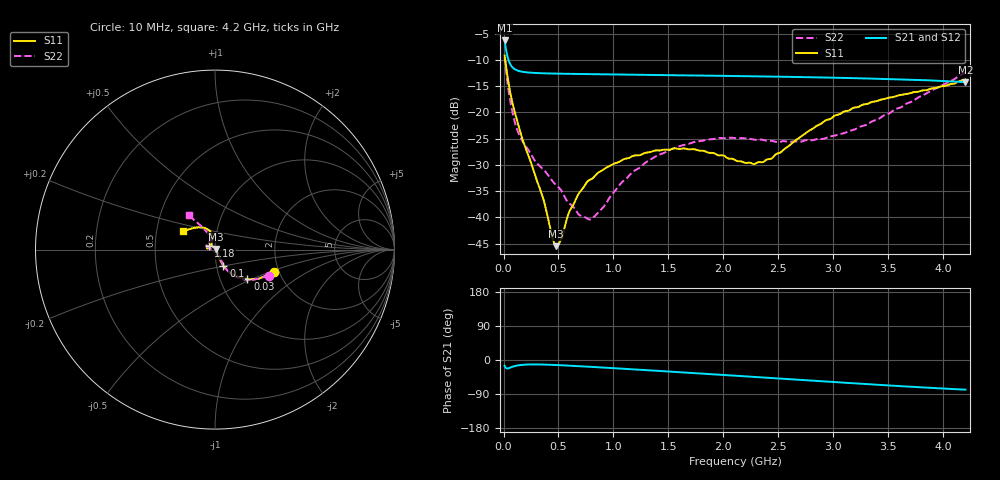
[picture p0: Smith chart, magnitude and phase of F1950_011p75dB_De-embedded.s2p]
! Integrated Device Technology
! Corporate Headquarters
! 6024 Silver Creek Valley Road
! San Jose, CA 95138  USA
! Phone:  1-408-284-8200
! Toll Free:  1-800-223-1366
! Webpage:  http://www.idt.com/
! Timing and RF Division
! 515 Groton Road, Suite 102
! Westford, MA 01886-6024
! Device:  F1950
! Description: 7-bit 0.25 dB Digital Step Attenuator
! Frequency:  150.0 -  4000.00 MHz
! Package:  4x4 mm Thin QFN Plastic Package: 24 pin
! Ports:  2 RF, 12 DC
!  Pin  1  = D0
!  Pin  2  = VDD
!  Pin  3  = Vmode
!  Pin  4  = GND
!  Pin  5  = RF1  =  Port 1
!  Pin  6  = GND
!  Pin  7  = GND
!  Pin  8  = GND
!  Pin  9  = GND
!  Pin 10  = GND
!  Pin 11  = GND
!  Pin 12  = GND
!  Pin 13  = GND
!  Pin 14  = RF2  =  Port 2
!  Pin 15  = GND
!  Pin 16  = LE
!  Pin 17  = CLK
!  Pin 18  = DATE
!  Pin 19  = D6
!  Pin 20  = D5
!  Pin 21  = D4
!  Pin 22  = D3
!  Pin 23  = D2
!  Pin 24  = D1
! State:  47
! Atten State:  11.75 dB
! Voltage:  +5.00 Volts
! Current:  Not Measured mA
! Data:  The device was measured on a the F195X evaluation board which has
!  individual transmission lines to the RF pins.  Data was collected
!  using a calibrated network analyzer.  The evaluation board was
!  de-embedded using a TRL calibration technique.
!  The reference plane is the edge of the package pin.
! Misc:  Board 2019
!  Action Tracker AT0250
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# GHz S dB R 50
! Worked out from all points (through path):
!   420 points, 10 MHz to 4.2 GHz, reference 50 ohm
!   highest |S21| = -6.29 dB at 10 MHz (marker M1); lowest = -14.2 dB at 4.2 GHz (marker M2)
!   group delay of S21, straight-line fit = 47.6 ps
!   lowest |S11| = -45.5 dB at 480 MHz (marker M3), VSWR 1.01, Z = 50.4 + j0.308 ohm
!   |S11| at or under -10 dB: 15.55 MHz to end of sweep
!   |S22| runs from -40.4 to -9.5 dB; largest |S21 - S12| = 0.00031
!   S11 on the Smith chart (normalised r, x): 10 MHz: 1.87, -0.54; 30 MHz: 1.35, -0.47; 100 MHz: 1.08, -0.20; 1.18 GHz: 0.93, +0.03; 4.2 GHz: 0.68, +0.15
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0.01  -9.13 -21.1  -6.29 -15.4  -6.29 -15.4  -9.48 -25.8
0.03  -12.21 -42.5  -8.80 -22.4  -8.80 -22.4  -13.36 -49.1
0.06  -16.12 -56.2  -10.77 -20.3  -10.77 -20.3  -17.67 -59.7
0.1  -19.77 -62.9  -11.74 -16.1  -11.74 -16.2  -21.65 -60.9
0.15  -23.57 -63.5  -12.16 -13.4  -12.16 -13.4  -24.58 -61.2
0.27  -30.83 -54.9  -12.47 -11.7  -12.47 -11.7  -28.69 -60.3
0.36  -36.37 -40.1  -12.55 -12.0  -12.55 -12.0  -30.82 -61.5
0.45  -44.24 0.8  -12.60 -12.9  -12.60 -12.9  -33.22 -63.4
0.48  -45.48 35.0  -12.61 -13.3  -12.61 -13.3  -33.90 -66.8
0.52  -44.33 72.4  -12.62 -13.8  -12.62 -13.8  -34.72 -67.7
0.6  -38.81 106.5  -12.65 -15.0  -12.65 -15.0  -37.37 -78.7
0.71  -34.78 121.3  -12.68 -16.7  -12.68 -16.7  -39.75 -102.2
0.82  -32.37 130.0  -12.72 -18.5  -12.72 -18.5  -39.98 -139.8
1.18  -28.27 152.4  -12.82 -24.6  -12.82 -24.6  -31.24 170.5
1.41  -27.24 163.8  -12.88 -28.7  -12.88 -28.7  -28.09 162.4
1.73  -27.00 172.2  -12.96 -34.5  -12.96 -34.5  -25.66 154.1
2.11  -29.12 162.4  -13.07 -41.5  -13.07 -41.5  -24.91 144.0
2.36  -29.45 132.3  -13.15 -46.1  -13.15 -46.1  -25.23 135.3
2.81  -23.13 101.4  -13.31 -54.5  -13.30 -54.5  -25.29 115.3
3.1  -19.78 104.9  -13.43 -59.9  -13.43 -59.9  -23.93 110.4
3.51  -17.17 117.7  -13.64 -67.3  -13.64 -67.3  -20.16 113.4
4.2  -13.70 149.6  -14.23 -78.2  -14.23 -78.2  -12.37 127.5
